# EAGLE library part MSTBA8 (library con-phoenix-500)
PHOENIX
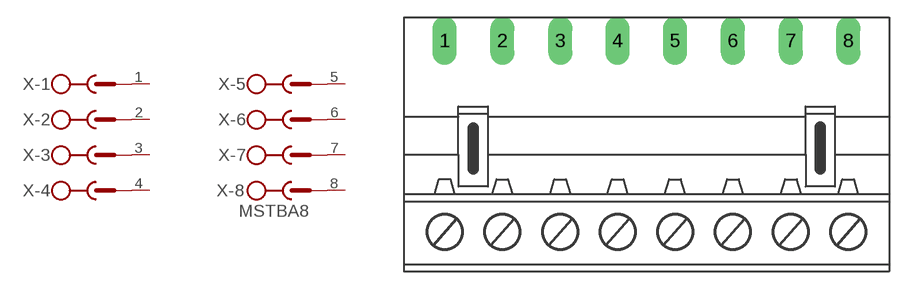
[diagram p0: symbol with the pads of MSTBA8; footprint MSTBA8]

Designator prefix X; gates -1=SK -2=SK -3=SK -4=SK -5=SK -6=SK -7=SK -8=SK+V

## MSTBA8 (OC_FARNELL: unknown; OC_NEWARK: unknown)  [MSTBA8]
1  -1:SK  pas
2  -2:SK  pas
3  -3:SK  pas
4  -4:SK  pas
5  -5:SK  pas
6  -6:SK  pas
7  -7:SK  pas
8  -8:SK  pas

## Footprint MSTBA8 (pad centres in mm)
PHOENIX
drill 1.397 long: 1 -17.462,7.62; 2 -12.459,7.62; 3 -7.429,7.62; 4 -2.451,7.62; 5 2.527,7.62; 6 7.556,7.62; 7 12.586,7.62; 8 17.564,7.62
